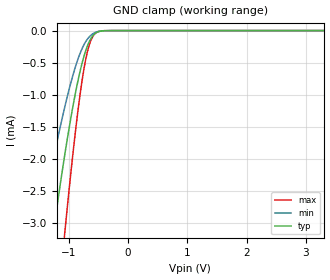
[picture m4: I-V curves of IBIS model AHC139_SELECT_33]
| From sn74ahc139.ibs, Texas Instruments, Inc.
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[Model]   AHC139_SELECT_33
Model_type  Input
Vinl=0.9
Vinh=2.1
| variable   typ   min   max
C_comp   0.75pF   0.55pF   0.87pF
[Temperature Range]   40   100   -40
| Ambient temperature   25   85   -40
[Voltage range]   3.3   3   3.6
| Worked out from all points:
|   GND clamp passes 1 mA (typ) near -0.89 V on its own axis
[GND Clamp]
| AHC139_SELECT_33
|   Voltage   I(typ)   I(min)   I(max)
-5.5V     -44.85mA   -29.94mA   -57.22mA
-1.52V    -5.007mA   -3.243mA   -7.831mA
-1.49V    -4.782mA   -3.093mA   -7.502mA
-1.265V   -3.18mA    -2.024mA   -5.105mA
-1.24V    -3.013mA   -1.912mA   -4.849mA
-1.065V   -1.918mA   -1.18mA    -3.125mA
-890mV    -985.3uA   -570.7uA   -1.59mA
-825mV    -697.7uA   -392.9uA   -1.103mA
-755mV    -436.9uA   -240.6uA   -657.7uA
-650mV    -163.1uA   -93.54uA   -211.3uA
-535mV    -31.97uA   -22.37uA   -31.27uA
3.3V      4.502nA    731.3pA    21.74nA
